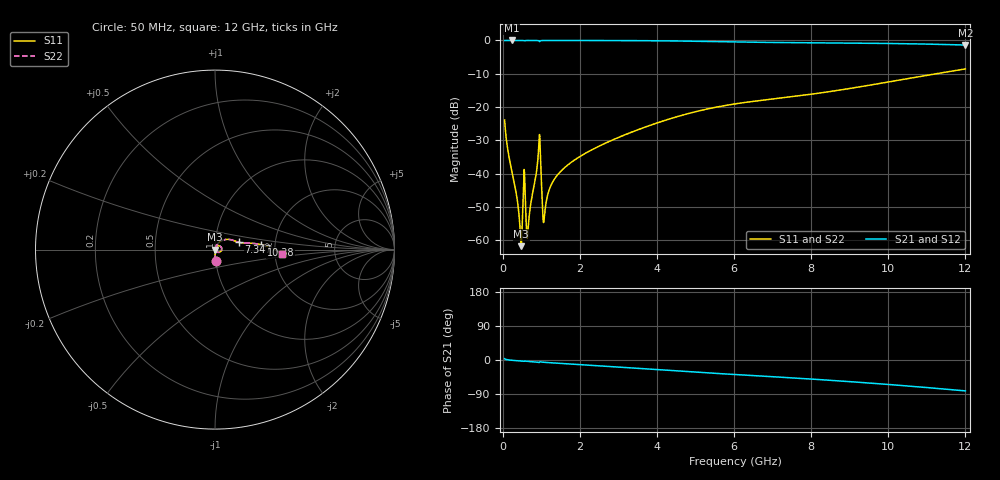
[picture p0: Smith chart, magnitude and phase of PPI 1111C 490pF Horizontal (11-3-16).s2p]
# MHz S MA R 50
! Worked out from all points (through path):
!   1601 points, 50 MHz to 12 GHz, reference 50 ohm
!   highest |S21| = 0.00 dB at 229.2 MHz (marker M1); lowest = -1.4 dB at 12 GHz (marker M2)
!   group delay of S21, straight-line fit = 18.4 ps
!   lowest |S11| = -61.7 dB at 483.2 MHz (marker M3), VSWR 1.00, Z = 50.1 - j0.00121 ohm
!   |S11| at or under -10 dB: start of sweep to 11.24 GHz
!   |S22| runs from -61.7 to -8.5 dB; largest |S21 - S12| = 0
!   S11 on the Smith chart (normalised r, x): 50 MHz: 1.00, -0.13; 7.347 GHz: 1.30, +0.11; 10.38 GHz: 1.69, +0.10; 12 GHz: 2.19, -0.11
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50  0.06393 -86.4  0.9977 3.4  0.9977 3.4  0.06393 -86.4
229.25  0.01153 -88.4  0.9995 -0.6  0.9995 -0.6  0.01153 -88.4
356.2188  0.004909 -85.3  0.9994 -1.7  0.9994 -1.7  0.004909 -85.3
438.375  0.001924 -72.4  0.9993 -2.3  0.9993 -2.3  0.001924 -72.4
483.1875  0.0008207 -0.8  0.9992 -2.7  0.9992 -2.7  0.0008207 -0.8
557.875  0.01163 7.7  0.9885 -3.2  0.9885 -3.2  0.01163 7.7
640.0312  0.001107 18.8  0.9989 -3.6  0.9989 -3.6  0.001107 18.8
669.9062  0.001807 55.4  0.999 -3.8  0.999 -3.8  0.001807 55.4
931.3125  0.02351 58.0  0.9896 -6.4  0.9896 -6.4  0.02351 58.0
976.125  0.02144 -44.6  0.9834 -4.6  0.9834 -4.6  0.02144 -44.6
1050.812  0.001985 -12.1  0.998 -5.8  0.998 -5.8  0.001985 -12.1
1088.156  0.002476 47.3  0.9985 -6.2  0.9985 -6.2  0.002476 47.3
1200.188  0.005624 71.6  0.9988 -7.0  0.9988 -7.0  0.005624 71.6
1349.562  0.008446 74.7  0.9988 -8.0  0.9988 -8.0  0.008446 74.7
2044.156  0.01876 73.0  0.9982 -12.4  0.9982 -12.4  0.01876 73.0
4038.312  0.05875 54.7  0.988 -25.4  0.988 -25.4  0.05875 54.7
6025  0.1117 28.0  0.9496 -38.3  0.9496 -38.3  0.1117 28.0
7346.969  0.1398 16.7  0.9282 -46.2  0.9282 -46.2  0.1398 16.7
8019.156  0.1566 13.9  0.9217 -50.4  0.9217 -50.4  0.1566 13.9
10013.31  0.2387 7.6  0.9005 -64.7  0.9005 -64.7  0.2387 7.6
10379.28  0.2598 6.0  0.8944 -67.6  0.8944 -67.6  0.2598 6.0
12000  0.3737 -3.5  0.8528 -81.5  0.8528 -81.5  0.3737 -3.5
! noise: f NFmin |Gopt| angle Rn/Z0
50  0.0003509  0.8585  0.3212  0.0005308
1372  0.003772  0.6756  7.584  0.002233
2701  0.008172  0.7035  14.82  0.005319
4031  0.01928  0.8048  22.01  0.01979
5360  0.03904  0.8703  29.02  0.06075
6682  0.05853  0.8939  35.73  0.109
8012  0.06982  0.8967  42.22  0.1285
9341  0.07652  0.8943  48.41  0.1314
1.067e+04  0.08252  0.8926  54.31  0.1327
1.2e+04  0.08932  0.8932  59.9  0.137
